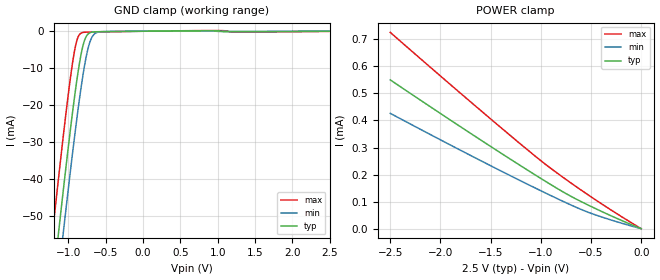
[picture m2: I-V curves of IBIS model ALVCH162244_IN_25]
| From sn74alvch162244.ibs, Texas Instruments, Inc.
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[Model]   ALVCH162244_IN_25
Model_type  Input
Vinl=0.7
Vinh=1.7
| variable   typ   min   max
C_comp   5.19pF   4.19pF   6.27pF
[Temperature Range]   40   100   -40
| Ambient temperature   25   85   -40
[Voltage range]   2.5   2.3   2.7
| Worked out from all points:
|   GND clamp passes 1 mA (typ) near -0.75 V on its own axis
[GND Clamp]
| ALVCH162244_IN_25
|   Voltage   I(typ)   I(min)   I(max)
-2.5V     -319.5mA   -330.1mA   -306.3mA
-1.23V    -72.41mA   -83.9mA    -57.69mA
-1.2V     -66.83mA   -78.33mA   -52.08mA
-1.13V    -53.97mA   -65.47mA   -39.2mA
-1.07V    -43.18mA   -54.64mA   -28.49mA
-925mV    -18.79mA   -29.65mA   -6.062mA
-880mV    -12.23mA   -22.5mA    -2.049mA
-830mV    -6.17mA    -15.15mA   -505.2uA
-780mV    -2.23mA    -8.823mA   -271.3uA
-720mV    -496.1uA   -3.399mA   -227.6uA
-595mV    -130.6uA   -218.3uA   -183.1uA
2.5V      6.664pA    20.75uA    -42.68uA
[POWER Clamp]
| ALVCH162244_IN_25
|   Voltage   I(typ)   I(min)   I(max)
-2.5V     550.2uA    426.5uA    725.8uA
-1.6V     328.2uA    251.7uA    437.3uA
-970mV    178.8uA    134.8uA    242.7uA
-735mV    126.7uA    93.49uA    178.2uA
-520mV    85.76uA    59.48uA    122.8uA
-280mV    44.19uA    29.72uA    64.16uA
-31.15fV  6.664pA    10.41pA    6.889pA
